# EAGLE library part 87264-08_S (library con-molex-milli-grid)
RECEPTACAL
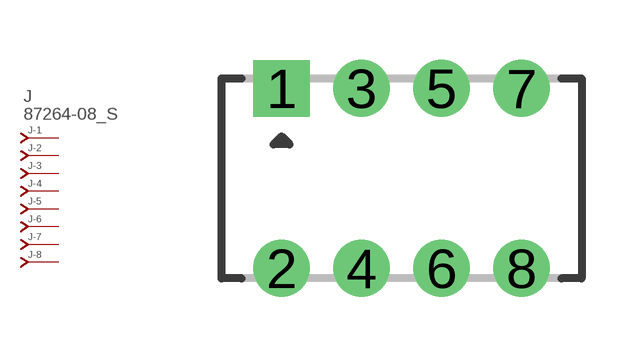
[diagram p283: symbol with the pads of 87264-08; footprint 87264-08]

Designator prefix J; gates -1=J-NV -2=J-N -3=J-N -4=J-N -5=J-N -6=J-N -7=J-N -8=J-N

## 87264-08_S  [87264-08]
1  -1:J  pas
2  -2:J  pas
3  -3:J  pas
4  -4:J  pas
5  -5:J  pas
6  -6:J  pas
7  -7:J  pas
8  -8:J  pas

## Footprint 87264-08 (pad centres in mm)
RECEPTACAL Dual Row, Side Entry
drill 0.914 square: 1 -3,2.25
drill 0.914: 2 -3,-2.25; 3 -1,2.25; 4 -1,-2.25; 5 1,2.25; 6 1,-2.25; 7 3,2.25; 8 3,-2.25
